(* Logix 5000 AddOnInstructionDefinition export AMCI_3601_AOP_Min_Registration_Distance; software revision 20.03 *)

ADD_ON_INSTRUCTION AMCI_3601_AOP_Min_Registration_Distance   (* revision 0.0, vendor AMCI, ExecuteEnableInFalse *)
// Revision note:
// 3/2020: Version 0 is the initial release
VAR_INPUT
   Axis_Status_Bits : INT; {required}
   Target_Position : DINT; {required}
END_VAR
VAR_OUTPUT
   EN : BOOL; {access Read Only, visible}
   ER : BOOL; {access Read Only, visible}
END_VAR
VAR_IN_OUT
   AMCI_3601_output_data : AM:1769_3601:O:0; {required}
END_VAR
VAR
   Upper_Result_X_1000 : DINT;
   command_data_block : INT[10];
        [0]   // Command Bits MSW
        [1]   // Command Bits LSW
        [2]   // Upper Target Position
        [3]   // Lower Target Position
        [4]   // Upper Programmed Speed
        [5]   // Lower Programmed Speed
END_VAR

ROUTINE EnableInFalse   (* ladder *)
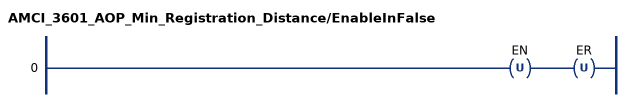
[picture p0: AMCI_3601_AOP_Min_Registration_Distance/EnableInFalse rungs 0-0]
   0: OTU(EN)OTU(ER);
END_ROUTINE

ROUTINE Logic   (* ladder *)
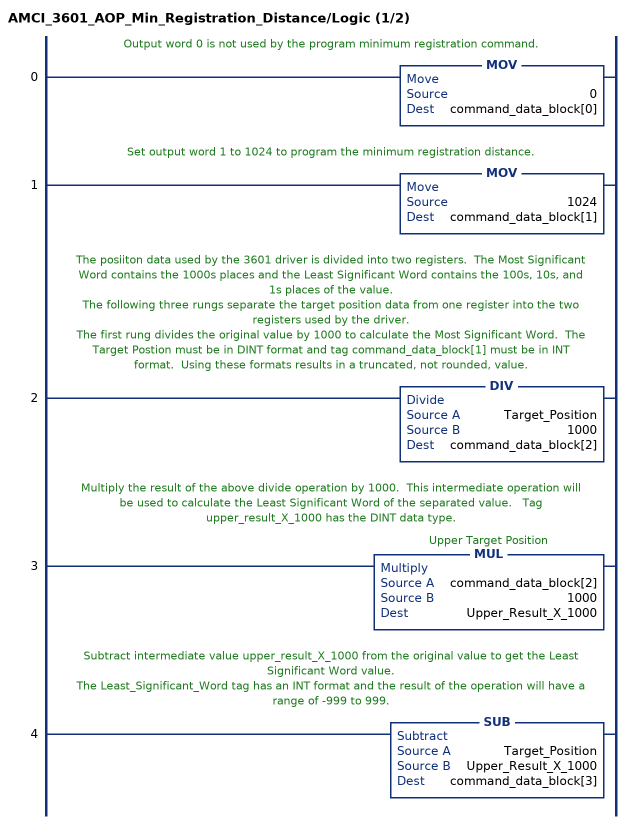
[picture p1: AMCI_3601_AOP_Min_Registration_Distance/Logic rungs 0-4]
   // Output word 0 is not used by the program minimum registration command.
   0: MOV(0,command_data_block[0]);
   // Set output word 1 to 1024 to program the minimum registration distance.
   1: MOV(1024,command_data_block[1]);
   // The posiiton data used by the 3601 driver is divided into two registers.  The Most Significant Word contains the 1000s places and the Least Significant Word contains the 100s, 10s, and 1s places of the value.
   // The following three rungs separate the target position data from one register into the two registers used by the driver.
   // The first rung divides the original value by 1000 to calculate the Most Significant Word.  The Target Postion must be in DINT format and tag command_data_block[1] must be in INT format.  Using these formats results in a truncated, not rounded, value.
   2: DIV(Target_Position,1000,command_data_block[2]);
   // Multiply the result of the above divide operation by 1000.  This intermediate operation will be used to calculate the Least Significant Word of the separated value.   Tag upper_result_X_1000 has the DINT data type.
   3: MUL(command_data_block[2],1000,Upper_Result_X_1000);
   // Subtract intermediate value upper_result_X_1000 from the original value to get the Least Significant Word value.
   // The Least_Significant_Word tag has an INT format and the result of the operation will have a range of -999 to 999.
   4: SUB(Target_Position,Upper_Result_X_1000,command_data_block[3]);
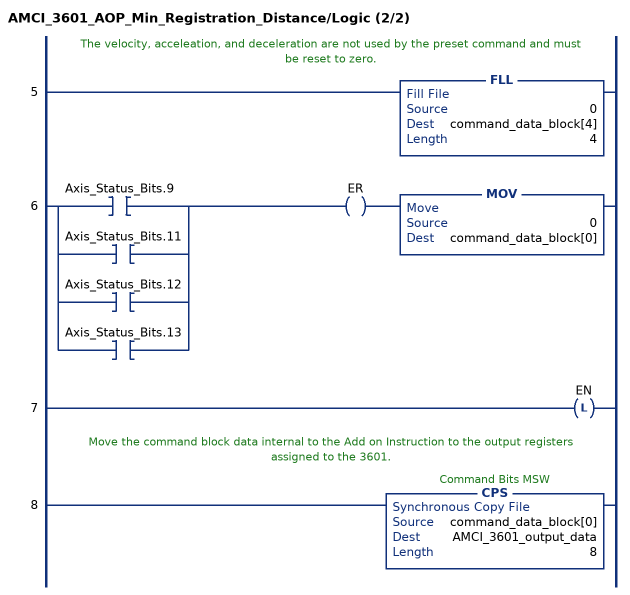
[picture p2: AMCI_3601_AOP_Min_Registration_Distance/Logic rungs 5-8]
   // The velocity, acceleation, and deceleration are not used by the preset command and must be reset to zero.
   5: FLL(0,command_data_block[4],4);
   6: [XIC(Axis_Status_Bits.9) ,XIC(Axis_Status_Bits.11) ,XIC(Axis_Status_Bits.12) ,XIC(Axis_Status_Bits.13) ]OTE(ER)MOV(0,command_data_block[0]);
   7: OTL(EN);
   // Move the command block data internal to the Add on Instruction to the output registers assigned to the 3601.
   8: CPS(command_data_block[0],AMCI_3601_output_data,8);
END_ROUTINE
END_ADD_ON_INSTRUCTION
